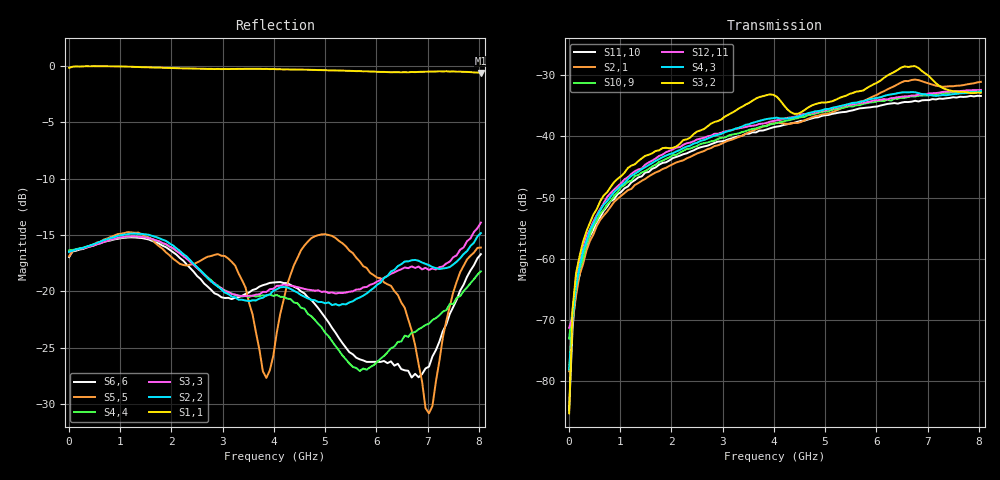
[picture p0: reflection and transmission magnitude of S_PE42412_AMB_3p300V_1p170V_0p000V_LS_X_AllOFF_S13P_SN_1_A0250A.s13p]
! Device ID: PE42412
! File Path: z:\PE42412\All_States_Off_PE42412\AMB\3p300\LS_X\PE42412_AMB_3p300V_1p170V_0p000V_LS_X_AllOFF_S13P_SN_1_A0250A.s13p
! Serial: 1
! Lot: A0250A
! Temp: AMB
! VDD: 3.300
! VSS: 0.000
! Control_Hi: 1.170
! Control_Lo: 0.000
! Logic State: LS_X_AllOFF
! Port 1:
! Port 2:
! Port 3:
! Port 4:
! Port 5:
! Port 6:
! Port 7:
! Port 8:
! Port 9:
! Port 10:
! Port 11:
! Port 12:
! Port 13:
! ThroughPath:1-2
! IDD: 0.0001071655
! ISS/IDD2: 1.262e-007
! IDMM3/IDD3: -2.002e-007
! Comment:
#  Hz  S  RI  R  50
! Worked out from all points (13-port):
!   120 points, 10 MHz to 8.037 GHz, reference 50 ohm
!   strongest paths, dB at 10 MHz, 2.034 GHz, 4.057 GHz, 6.08 GHz, 8.037 GHz:
!     S3,2: -85.2, -41.9, -33.5, -30.9, -32.9
!     S4,3: -78.1, -42.8, -37.0, -33.6, -32.6
!     S12,11: -71.3, -42.1, -37.4, -34.0, -32.4
!     S10,9: -73.0, -43.1, -37.8, -34.2, -32.5
!     S2,1: -78.4, -44.5, -37.8, -32.9, -31.1
!     S11,10: -84.7, -43.6, -38.4, -35.0, -33.4
!   lowest |S11| = -0.6 dB at 8.037 GHz (marker M1), VSWR 26.75, Z = 2.02 - j14.1 ohm
!   |S11| at or under -10 dB: nowhere
